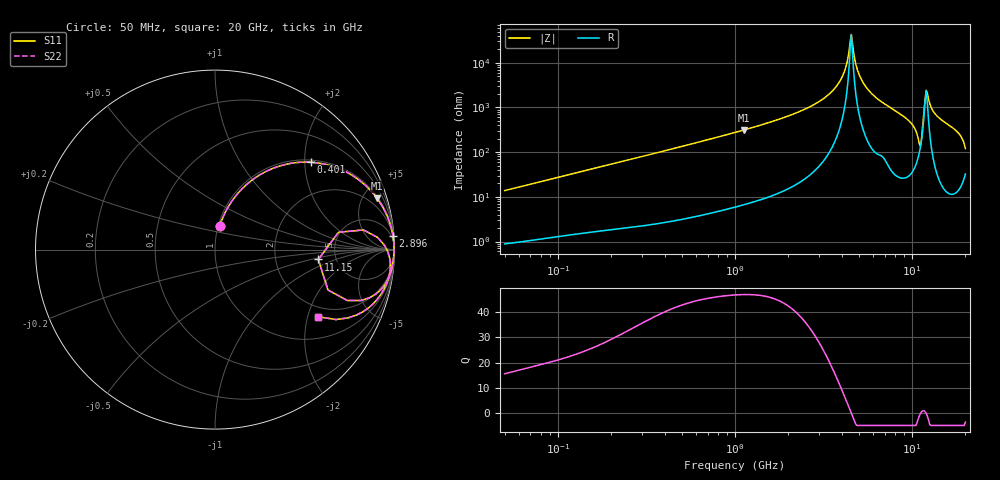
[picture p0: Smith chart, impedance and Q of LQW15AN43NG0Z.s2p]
!Murata Part Number: LQW15AN43NG0Z
!These Parameters are Measured in Series Mode Connection
!  o--[Z]--o
!Port1  Port2
!  o-------o
!Freq. Start=50[MHz] Stop=20[GHz], 401[Steps]
# Hz S RI R 50
!Freq.(Hz) S11(Real) S11(Imag) S21(Real) S21(Imag) S12(Real) S12(Imag) S22(Real) S22(Imag)
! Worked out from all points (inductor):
!   401 points, 50 MHz to 20 GHz, reference 50 ohm
!   read as one part in series: L = 43.6 nH near 51.52 MHz
!   highest Q = 47.1 at 1.127 GHz (marker M1), where L = 44.5 nH
!   self-resonance near 4.472 GHz
!   S11 on the Smith chart (normalised r, x): 50 MHz: 1.02, +0.28; 401 MHz: 1.05, +2.14; 2.896 GHz: 2, +25; 11.15 GHz: 3.63, -0.60; 20 GHz: 1.65, -2.33
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5e7  0.0269 0.1328  0.9731 -0.1328  0.9731 -0.1328  0.0269 0.1328
1.364002e8  0.1294 0.3155  0.8706 -0.3155  0.8706 -0.3155  0.1294 0.3155
3.721004e8  0.4976 0.4874  0.5024 -0.4874  0.5024 -0.4874  0.4976 0.4874
4.010383e8  0.5342 0.4865  0.4658 -0.4865  0.4658 -0.4865  0.5342 0.4865
1e9  0.8789 0.3158  0.1211 -0.3158  0.1211 -0.3158  0.8789 0.3158
1.127304e9  0.9036 0.2847  0.0964 -0.2847  0.0964 -0.2847  0.9036 0.2847
2.728004e9  0.9891 0.0893  0.0109 -0.0893  0.0109 -0.0893  0.9891 0.0893
2.896447e9  0.9911 0.0784  0.00888 -0.0784  0.00888 -0.0784  0.9911 0.0784
3.908127e9  0.997 0.0257  0.003 -0.0257  0.003 -0.0257  0.997 0.0257
4.149438e9  0.9975 0.0153  0.00255 -0.0153  0.00255 -0.0153  0.9975 0.0153
4.405649e9  0.9977 0.00496  0.00233 -0.00496  0.00233 -0.00496  0.9977 0.00496
4.539627e9  0.9977 -0.000262  0.00231 0.000262  0.00231 0.000262  0.9977 -0.000262
4.966507e9  0.9974 -0.0161  0.00263 0.0161  0.00263 0.0161  0.9974 -0.0161
5.352748e9  0.9966 -0.0297  0.00337 0.0297  0.00337 0.0297  0.9966 -0.0297
7.442007e9  0.9865 -0.0955  0.0135 0.0955  0.0135 0.0955  0.9865 -0.0955
1.050288e10  0.8621 -0.2677  0.1379 0.2677  0.1379 0.2677  0.8621 -0.2677
1.115139e10  0.5757 -0.0551  0.4243 0.0551  0.4243 0.0551  0.5757 -0.0551
1.183995e10  0.9432 0.0255  0.0568 -0.0255  0.0568 -0.0255  0.9432 0.0255
1.220001e10  0.9706 -0.0365  0.0294 0.0365  0.0294 0.0365  0.9706 -0.0365
1.354865e10  0.9721 -0.1368  0.0279 0.1368  0.0279 0.1368  0.9721 -0.1368
1.800918e10  0.879 -0.3039  0.121 0.3039  0.121 0.3039  0.879 -0.3039
2e10  0.5738 -0.3745  0.4262 0.3745  0.4262 0.3745  0.5738 -0.3745
